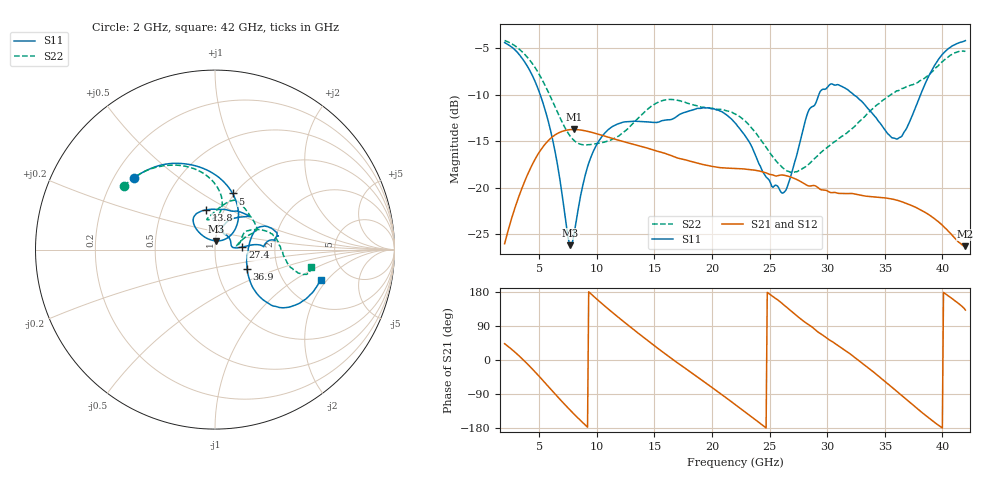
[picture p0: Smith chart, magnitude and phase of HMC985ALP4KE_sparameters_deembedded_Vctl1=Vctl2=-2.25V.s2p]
!s2p File: Measurements: S11, S21, S12, S22
# GHz S dB R 50.0
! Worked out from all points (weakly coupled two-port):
!   401 points, 2 GHz to 42 GHz, reference 50 ohm
!   highest |S21| = -13.74 dB at 8 GHz (marker M1); lowest = -26.3 dB at 42 GHz (marker M2)
!   lowest |S11| = -26.2 dB at 7.7 GHz (marker M3), VSWR 1.10, Z = 50.4 + j4.91 ohm
!   |S11| at or under -10 dB: 5.089 GHz to 29.28 GHz (24.19 GHz wide, 141 % of centre); 32.29 GHz to 38.11 GHz (5.813 GHz wide, 16.5 % of centre)
!   |S22| runs from -18.4 to -4.2 dB; largest |S21 - S12| = 0.00016
!   S11 on the Smith chart (normalised r, x): 2 GHz: 0.28, +0.35; 5 GHz: 0.98, +0.69; 13.8 GHz: 0.83, +0.39; 27.4 GHz: 1.36, +0.04; 36.9 GHz: 1.39, -0.32; 42 GHz: 3.19, -1.75
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2  -4.40 138.6  -26.03 43.1  -26.04 43.1  -4.17 145.0
3.5  -6.06 107.3  -20.08 3.9  -20.08 3.9  -5.37 119.5
5  -9.69 72.6  -16.20 -43.1  -16.20 -43.1  -7.81 95.3
6.2  -15.02 47.5  -14.49 -83.6  -14.49 -83.6  -10.81 82.4
7.7  -26.20 82.0  -13.76 -132.7  -13.77 -132.7  -14.47 85.9
8  -25.18 108.1  -13.74 -141.9  -13.75 -142.0  -14.89 89.1
8.7  -20.25 130.7  -13.82 -162.9  -13.82 -162.9  -15.37 96.9
10.6  -14.27 128.5  -14.43 144.9  -14.43 144.9  -15.12 105.0
13.8  -12.89 102.4  -15.54 66.0  -15.55 65.9  -12.27 81.7
15.4  -12.94 82.3  -16.14 28.5  -16.14 28.5  -10.78 71.1
19  -11.47 45.1  -17.45 -50.5  -17.45 -50.5  -11.31 44.8
22  -13.02 53.8  -17.93 -117.1  -17.94 -117.1  -12.07 24.3
24.5  -18.46 73.4  -18.33 -174.6  -18.34 -174.6  -15.29 21.2
26.1  -20.59 15.6  -18.64 149.0  -18.64 148.9  -17.81 12.6
27.4  -16.31 5.3  -19.15 115.7  -19.15 115.7  -18.28 8.3
28.7  -11.29 3.4  -19.79 86.8  -19.79 86.8  -17.11 13.7
31.1  -9.02 16.1  -20.62 34.9  -20.63 34.9  -14.64 29.6
33.3  -11.13 26.9  -20.90 -14.3  -20.90 -14.3  -12.31 27.2
35.4  -14.35 7.3  -21.17 -66.3  -21.17 -66.2  -10.12 18.5
36.9  -13.61 -31.2  -21.71 -104.6  -21.71 -104.6  -9.13 9.4
39.7  -6.14 -41.1  -23.71 -173.1  -23.71 -173.0  -6.82 -15.0
42  -4.19 -15.9  -26.29 131.8  -26.30 131.7  -5.30 -10.2
